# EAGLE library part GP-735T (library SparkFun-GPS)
ADH-tech GP-735 - Easy-to-use, Ultra-high performance, GPS Smart Antenna Module ADH-tech GP-735 is a slim, ultra-high performance, easy to use GPS smart antenna module designed with u-blox’s latest 7th generation single chip. This feature rich GPS module not only shortens the design efforts but also provides powerful functions. The compact design allows fast adoption and high yield production. The power control feature is very convenient to turn on/off power just via GPIO control pin. It’s especially useful to turn off power as the GPS function is not needed in the host applications. Datasheet SparkFun Products GPS Receiver - GP-735 (56 Channel) (GPS-13670)
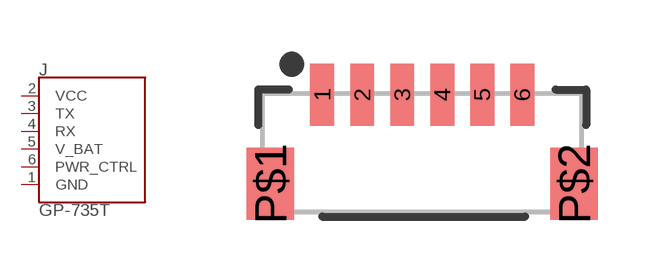
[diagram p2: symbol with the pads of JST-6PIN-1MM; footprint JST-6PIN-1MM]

Designator prefix J

## GP-735T-VERTICAL (PROD_ID: CONN-08249)  [JST-6PIN-1MM]
1  GND
2  VCC
3  TX
4  RX
5  V_BAT
6  PWR_CTRL

## Footprint JST-6PIN-1MM (pad centres in mm)
6-Pin Vertical JST Connector 1.0mm pitch JST-SH type Common interface for SparkFun GPS modules. Datasheet
smd 0.6 x 1.55: 1 -2.5,1.45; 2 -1.5,1.45; 3 -0.5,1.45; 4 0.5,1.45; 5 1.5,1.45; 6 2.5,1.45
smd 1.2 x 1.8: P$1 -3.8,-0.775; P$2 3.8,-0.775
